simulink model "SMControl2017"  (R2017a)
settings: Solver=VariableStepAuto  StartTime=0.0  StopTime=10.0  RelTol=1e-3
InitFcn:
  | initParams
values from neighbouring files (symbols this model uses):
  c = 8e-3    (= 0.008)    [initParams.m]
  g = 9.81    [initParams.m]
  K = 100    [initParams.m]
  L1 = 0.5    [initParams.m]
  lambda = 1    [initParams.m]
  m = 0.2    [initParams.m]
  phi = 0.01    [initParams.m]
  R = 10    [initParams.m]
  x0 = [0.1;0;0.3]    [initParams.m]
  x1d = 0.2    [initParams.m]

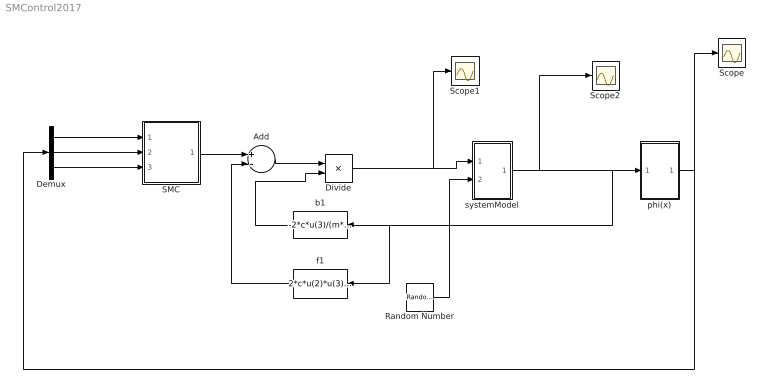
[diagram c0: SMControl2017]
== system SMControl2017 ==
  Add : Sum  Inputs=+-
  Demux : Demux  Outputs=3
  Divide : Product  Inputs=*/
  Random Number : RandomNumber  Variance=1e-2  SampleTime=0.01
  SMC : Subsystem
  Scope : Scope
  Scope1 : Scope
  Scope2 : Scope
  b1 : Fcn  Expr=-2*c*u(3)/(m*L1*u(1)^2)
  f1 : Fcn  Expr=2*c*u(2)*u(3)^2/(m*u(1)^3)-2*c*u(3)*(2*c*u(2)*u(3)/(L1*u(1)^2)-R*u(3)/L1)/(m*u(1)^2)
  phi(x) : Subsystem
  systemModel : Subsystem
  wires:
  SMC/1(v) -> Add/1
  b1/1 -> Divide/2
  f1/1 -> Add/2
  Add/1 -> Divide/1
  phi(x)/1(z) -> Scope/1, Demux/1
  Demux/2 -> SMC/2(ydot)
  Demux/3 -> SMC/3(yddot)
  Divide/1 -> Scope1/1, systemModel/1(u)
  systemModel/1(x) -> Scope2/1, f1/1, b1/1, phi(x)/1(x)
  Random Number/1 -> systemModel/2("d ")
  Demux/1 -> SMC/1(y)

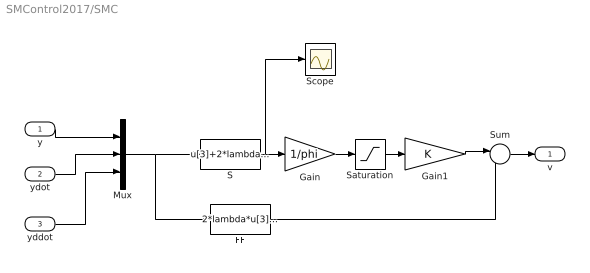
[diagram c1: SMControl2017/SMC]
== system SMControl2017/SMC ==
  y : Inport
  ydot : Inport  Port=2
  yddot : Inport  Port=3
  FF : Fcn  Expr=2*lambda*u[3]+lambda^2*u[2]
  Gain : Gain  Gain=1/phi
  Gain1 : Gain  Gain=K
  Mux : Mux  Inputs=3
  S : Fcn  Expr=u[3]+2*lambda*u[2]+lambda^2*u[1]
  Saturation : Saturate  UpperLimit=1  LowerLimit=-1
  Scope : Scope
  Sum : Sum  Inputs=|--
  v : Outport
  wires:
  S/1 -> Scope/1, Gain/1
  Gain/1 -> Saturation/1
  Saturation/1 -> Gain1/1
  Gain1/1 -> Sum/1
  FF/1 -> Sum/2
  Sum/1 -> v/1
  y/1 -> Mux/1
  ydot/1 -> Mux/2
  yddot/1 -> Mux/3
  Mux/1 -> S/1, FF/1

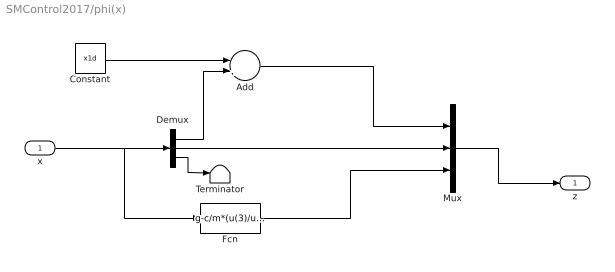
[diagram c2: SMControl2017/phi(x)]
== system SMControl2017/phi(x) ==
  x : Inport
  Add : Sum  Inputs=-+
  Constant : Constant  Value=x1d  SampleTime=0.01
  Demux : Demux  Outputs=3
  Fcn : Fcn  Expr=g-c/m*(u(3)/u(1))^2
  Mux : Mux  Inputs=3
  Terminator : Terminator
  z : Outport
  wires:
  Fcn/1 -> Mux/3
  x/1 -> Fcn/1, Demux/1
  Demux/1 -> Add/2
  Demux/3 -> Terminator/1
  Mux/1 -> z/1
  Constant/1 -> Add/1
  Add/1 -> Mux/1
  Demux/2 -> Mux/2

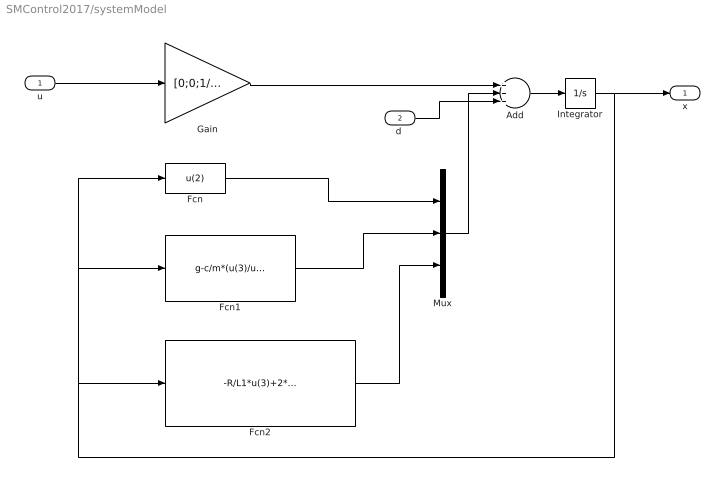
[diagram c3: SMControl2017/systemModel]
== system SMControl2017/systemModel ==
  u : Inport
  "d " : Inport  Port=2
  Add : Sum  Inputs=+++
  Fcn : Fcn  Expr=u(2)
  Fcn1 : Fcn  Expr=g-c/m*(u(3)/u(1))^2
  Fcn2 : Fcn  Expr=-R/L1*u(3)+2*c/L1*(u(2)*u(3)/(u(1))^2)
  Gain : Gain  Gain=[0;0;1/L1]  Multiplication=Matrix(K*u) (u vector)
  Integrator : Integrator  InitialCondition=x0
  Mux : Mux  Inputs=3
  x : Outport
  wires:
  Integrator/1 -> x/1, Fcn/1, Fcn1/1, Fcn2/1
  Gain/1 -> Add/1
  Fcn/1 -> Mux/1
  Fcn1/1 -> Mux/2
  Mux/1 -> Add/2
  Fcn2/1 -> Mux/3
  u/1 -> Gain/1
  Add/1 -> Integrator/1
  "d "/1 -> Add/3
